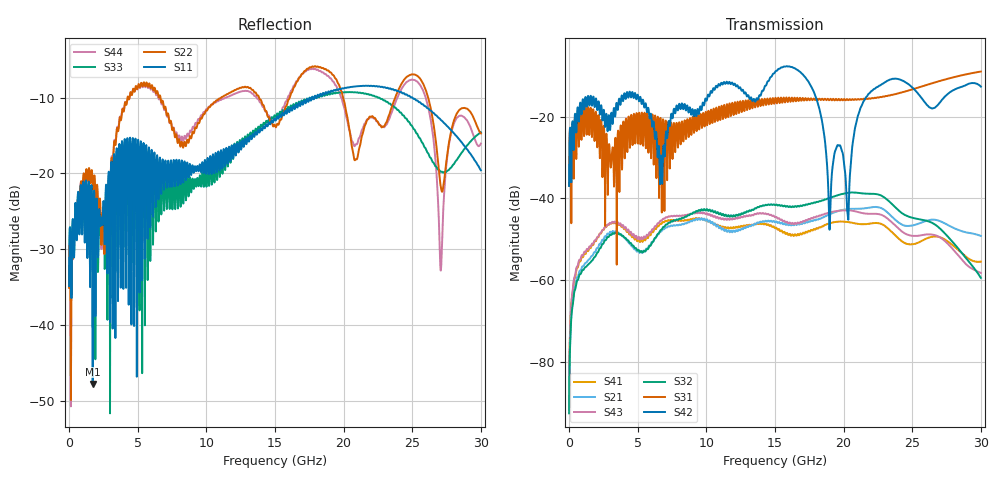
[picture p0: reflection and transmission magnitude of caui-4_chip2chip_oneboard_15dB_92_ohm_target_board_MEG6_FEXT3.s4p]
! Touchstone file from project caui-4_chip2chip_oneboard
! Exported from Circuit Design 8.0.0
! Variables:
!  $ModelNames_Index = 0
!  $ModelNames_Index1 = 0
!  $ModelNames_Index2 = 0
!  $ModelNames_Index3 = 0
!  $ModelNames_Index4 = 0
!  $ModelNames_Index5 = 0
!  Lbo = 0.5in
!  Lmain = 16in
!  lcap = 0.25in
# GHZ S MA R 50.000000
! Modal data exported
! Port[1] = Port1
! Port[2] = Port2
! Port[3] = Port3
! Port[4] = Port4
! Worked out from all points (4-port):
!   3000 points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, 10 MHz to 30 GHz, reference 50 ohm
!   strongest paths, dB at 10 MHz, 7.51 GHz, 15.01 GHz, 22.51 GHz, 30 GHz:
!     S42: -36.9, -20.0, -9.0, -12.6, -12.6
!     S31: -36.9, -26.8, -15.7, -15.3, -8.9
!     S32: -92.6, -45.6, -41.6, -39.0, -59.5
!     S43: -89.2, -44.3, -44.6, -43.8, -58.3
!     S21: -91.8, -46.7, -45.9, -42.1, -49.2
!     S41: -89.5, -45.4, -47.3, -46.0, -55.5
!   lowest |S11| = -47.8 dB at 1.73 GHz (marker M1), VSWR 1.01, Z = 50.2 + j0.335 ohm
!   |S11| at or under -10 dB: start of sweep to 17.69 GHz; 17.76 GHz to 17.87 GHz (107.7 MHz wide, 0.605 % of centre); 25.01 GHz to end of sweep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
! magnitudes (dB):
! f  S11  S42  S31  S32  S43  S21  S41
! 10 MHz  -34.9  -36.9  -36.9  -92.6  -89.2  -91.8  -89.5
! 1.73 GHz  -47.8  -15.9  -19.4  -55.1  -51.0  -53.9  -51.3
! 6.71 GHz  -22.6  -29.5  -23.7  -47.7  -45.5  -48.1  -46.3
! 16.33 GHz  -11.1  -8.0  -16.2  -42.0  -46.2  -46.4  -49.0
! 20.3 GHz  -8.7  -43.9  -15.8  -38.6  -42.9  -42.6  -45.8
! 22.09 GHz  -8.5  -13.6  -15.4  -38.9  -43.8  -42.1  -46.1
! 30 GHz  -19.6  -12.6  -8.9  -59.5  -58.3  -49.2  -55.5
